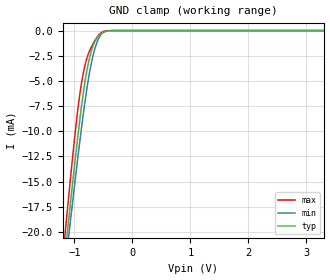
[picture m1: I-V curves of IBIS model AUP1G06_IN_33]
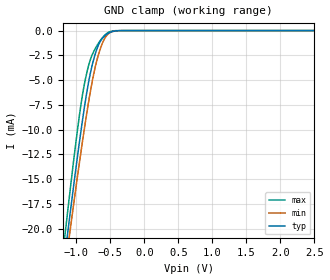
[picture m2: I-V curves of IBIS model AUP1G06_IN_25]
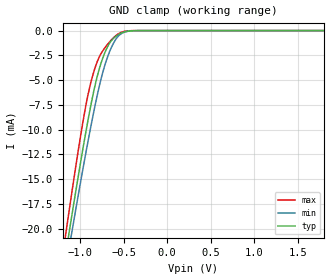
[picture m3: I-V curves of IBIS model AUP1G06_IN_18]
| TEXAS INSTRUMENTS INCORPORATED
| Standard Linear and Logic Group
| IBIS Model of SN74AUP1G06
| Low-Power Single Inverter Buffer/Driver with Open-Drain Output
| This file contains package information for the following:
|  SON 6-pin (DRY) package as [Component] AUP1G06_DRY
|  SON 6-pin (DSF) package as [Component] AUP1G06_DSF
|  SOT 5-pin (DCK) package as [Component] AUP1G06_DCK
|  SOT 5-pin (DBV) package as [Component] AUP1G06_DBV
| This device can be powered at the following Vccs:
|  3.3 volt Vcc
|  2.5 volt Vcc
|  1.8 volt Vcc
|  1.5 volt Vcc
|  1.2 volt Vcc
|  0.8 volt Vcc
| This file provides unique models under the [Model Selector] for each Vcc.
| For operation at a specific Vcc, select the appropriate model after each
| [Model Selector] keyword.
[IBIS Ver]   3.2
[Comment char]  |_char
[File Name]   sn74aup1g06.ibs
[File Rev]   1.1 | x_die
[Date]   April 30,2004
[Source]   Data creted from TI-SPICE simulations at TI-SLL.
[Notes]   The following is an IBIS list for the AUP1G06.
   Please contact sllibis@ti.com with questions and
   comments concerning SLL IBIS models.
   - FILE REV HISTORY
   - 1.1 Release IBIS file on 05/04/04
   - Power clamp data deleted as there is no power-clamp diode.
[Disclaimer] Property of Texas Instruments Incorporated.  Unauthorized
   reproduction and/or distribution is strictly prohibited.
   This product is protected under copyright law.
   Created  2003, (C) Copyright  2003, Texas Instruments
   Incorporated, All Rights Reserved
   UNLESS THERE IS A SIGNED, WRITTEN AGREEMENT TO THE
   CONTRARY, TEXAS INSTRUMENTS (TI) IS PROVIDING THE IBIS
   MODELS  AND WITHOUT ANY WARRANTY, EXPRESSED OR
   IMPLIED.  TI assumes no liability for:
   1) the accuracy of the IBIS models provided to your
   company;
   2) the proper functioning of these IBIS Models in your
   design or for any resulting applications; or
   3) infringement of patents, copyrights or intellectual
   property rights resulting from your use of these IBIS
   models.
   TI provides IBIS Models as a service to our customers.
   You and your company shall not distribute, sell or give
   these models to anyone else without prior written
   permission from TI.
   TI reserves the right to make changes to our products or
   to discontinue any semiconductor product or service
   without notice, and advises our customers to obtain the
   latest version of relevant information to verify, before
   placing orders, that the information being relied on is
   current.
   Please be aware that your receipt and use of the IBIS
   information provided shall serve as acceptance of these
   terms and conditions.  If you do not accept these terms,
   you should return or destroy the IBIS models and any
   other accompanying information immediately.
| Component AUP1G06_DRY 6-pin SON
[Component]   AUP1G06_DRY
[Manufacturer]   Texas Instruments, Inc.
[Package]
|   typ   min   max
R_pkg   2.61E-02   1.03E-03   4.37E-02
L_pkg   2.94E-10   1.45E-11   5.00E-10
C_pkg   1.01E-13   7.41E-14   1.18E-13
[Pin]   signal_name   model_name   R_pin   L_pin   C_pin
1   NC   NC   1.03E-03   1.46E-11   7.41E-14
2   A   AUP1G06_IN   3.24E-02   3.52E-10   1.09E-13
3   GND   GND   3.93E-02   4.44E-10   1.14E-13
4   Y   AUP1G06_OUT   3.93E-02   4.39E-10   1.14E-13
5   NC   NC   1.03E-03   1.45E-11   7.65E-14
6   VCC   POWER   4.37E-02   5.00E-10   1.18E-13
| Component AUP1G06_DSF 6-pin SON
[Component]   AUP1G06_DSF
[Manufacturer]   Texas Instruments, Inc.
[Package]
|   typ   min   max
R_pkg   2.24E-02   1.03E-03   3.70E-02
L_pkg   2.53E-10   1.77E-11   4.23E-10
C_pkg   9.79E-14   7.41E-14   1.13E-13
[Pin]   signal_name   model_name   R_pin   L_pin   C_pin
1   NC   NC   3.06E-03   1.77E-11   7.41E-14
2   A   AUP1G06_IN   2.77E-02   3.06E-10   1.06E-13
3   GND   GND   3.21E-02   3.60E-10   1.08E-13
4   Y   AUP1G06_OUT   3.35E-02   3.75E-10   1.10E-13
5   NC   NC   1.03E-03   3.45E-11   7.65E-14
6   VCC   POWER   3.70E-02   4.23E-10   1.13E-13
| Component AUP1G06_DCK 5-pin SOT
[Component]   AUP1G06_DCK
[Manufacturer]   Texas Instruments, Inc.
[Package]
|   typ   min   max
R_pkg   2.000e-02   1.700e-02   2.500e-02
L_pkg   9.980e-10   8.810e-10   1.069e-09
C_pkg   1.460e-13   1.180e-13   2.050e-13
[Pin]   signal_name   model_name   R_pin   L_pin   C_pin
1   NC   NC   1.900e-02   1.069e-09   1.620e-13
2   A   AUP1G06_IN   1.800e-02   8.810e-10   1.210e-13
3   GND   GND   1.700e-02   1.031e-09   2.050e-13
4   Y   AUP1G06_OUT   2.000e-02   9.600e-10   1.240e-13
5   VCC   POWER   2.500e-02   1.049e-09   1.180e-13
| Component AUP1G06_DBV 5-pin SOT
[Component]   AUP1G06_DBV
[Manufacturer]   Texas Instruments, Inc.
[Package]
|   typ   min   max
R_pkg   2.500e-02   2.100e-02   2.900e-02
L_pkg   1.529e-09   1.312e-09   1.906e-09
C_pkg   1.560e-13   1.100e-13   2.400e-13
[Pin]   signal_name   model_name   R_pin   L_pin   C_pin
1   NC   NC   2.100e-02   1.511e-09   1.440e-13
2   A   AUP1G06_IN   2.300e-02   1.312e-09   1.380e-13
3   GND   GND   2.900e-02   1.906e-09   2.400e-13
4   Y   AUP1G06_OUT   2.600e-02   1.541e-09   1.500e-13
5   VCC   POWER   2.500e-02   1.374e-09   1.100e-13
| Model AUP1G06_IN
[Model Selector]   AUP1G06_IN
AUP1G06_IN_33   3.3 volt Vcc
AUP1G06_IN_25   2.5 volt Vcc
AUP1G06_IN_18   1.8 volt Vcc
AUP1G06_IN_15   1.5 volt Vcc
AUP1G06_IN_12   1.2 volt Vcc
AUP1G06_IN_08   0.8 volt Vcc
| Model AUP1G06_OUT
[Model Selector]   AUP1G06_OUT
AUP1G06_OUT_33   3.3 volt Vcc
AUP1G06_OUT_25   2.5 volt Vcc
AUP1G06_OUT_18   1.8 volt Vcc
AUP1G06_OUT_15   1.5 volt Vcc
AUP1G06_OUT_12   1.2 volt Vcc
AUP1G06_OUT_08   0.8 volt Vcc
| Models and submodels in the file (12): AUP1G06_IN_33 (Input), AUP1G06_IN_25 (Input), AUP1G06_IN_18 (Input), AUP1G06_IN_15 (Input), AUP1G06_IN_12 (Input), AUP1G06_IN_08 (Input), AUP1G06_OUT_33 (Open_drain), AUP1G06_OUT_25 (Open_drain), AUP1G06_OUT_18 (Open_drain), AUP1G06_OUT_15 (Open_drain), AUP1G06_OUT_12 (Open_drain), AUP1G06_OUT_08 (Open_drain)
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[Model]   AUP1G06_IN_33
Model_type  Input
Vinl=0.9
Vinh=2
| variable   typ   min   max
C_comp   1.41pF   1.15pF   1.78pF
[Temperature Range]   40   100   -40
| Ambient temperature   25   85   -40
[Voltage range]   3.3   3   3.6
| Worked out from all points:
|   GND clamp passes 1 mA (typ) near -0.64 V on its own axis
[GND Clamp]
| AUP1G06_IN_33
|   Voltage   I(typ)   I(min)   I(max)
-3.6V     -171.6mA   -163.5mA   -181.1mA
-1.16V    -22.22mA   -23.69mA   -20.18mA
-1.11V    -19.45mA   -21.09mA   -17.19mA
-1.085V   -18.08mA   -19.81mA   -15.71mA
-940mV    -10.5mA    -12.6mA    -7.822mA
-890mV    -8.117mA   -10.26mA   -5.698mA
-835mV    -5.768mA   -7.825mA   -3.925mA
-755mV    -3.153mA   -4.717mA   -2.255mA
-675mV    -1.463mA   -2.419mA   -1.277mA
-595mV    -617.7uA   -945.8uA   -546.7uA
-515mV    -215.4uA   -248.8uA   -134.4uA
3.3V      132.2pA    540.4pA    36.28pA
[Model]   AUP1G06_IN_25
Model_type  Input
Vinl=0.7
Vinh=1.6
| variable   typ   min   max
C_comp   1.44pF   1.20pF   1.77pF
[Temperature Range]   40   100   -40
| Ambient temperature   25   85   -40
[Voltage range]   2.5   2.3   2.7
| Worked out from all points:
|   GND clamp passes 1 mA (typ) near -0.64 V on its own axis
[GND Clamp]
| AUP1G06_IN_25
|   Voltage   I(typ)   I(min)   I(max)
-3.6V     -171.6mA   -163.5mA   -181.1mA
-1.165V   -22.5mA    -23.95mA   -20.48mA
-1.115V   -19.72mA   -21.35mA   -17.49mA
-1.09V    -18.36mA   -20.06mA   -16.01mA
-945mV    -10.75mA   -12.84mA   -8.061mA
-890mV    -8.117mA   -10.26mA   -5.698mA
-835mV    -5.768mA   -7.825mA   -3.925mA
-760mV    -3.287mA   -4.89mA    -2.329mA
-675mV    -1.463mA   -2.419mA   -1.277mA
-595mV    -617.7uA   -945.8uA   -546.7uA
-520mV    -233.1uA   -272.6uA   -149.9uA
2.5V      104.3pA    491.9pA    26.71pA
[Model]   AUP1G06_IN_18
Model_type  Input
Vinl=0.6825
Vinh=1.0725
| variable   typ   min   max
C_comp   1.49pF   1.27pF   1.76pF
[Temperature Range]   40   100   -40
| Ambient temperature   25   85   -40
[Voltage range]   1.8   1.65   1.95
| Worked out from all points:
|   GND clamp passes 1 mA (typ) near -0.64 V on its own axis
[GND Clamp]
| AUP1G06_IN_18
|   Voltage   I(typ)   I(min)   I(max)
-3.6V     -171.6mA   -163.5mA   -181.1mA
-1.16V    -22.22mA   -23.69mA   -20.18mA
-1.135V   -20.83mA   -22.39mA   -18.68mA
-1.11V    -19.45mA   -21.09mA   -17.19mA
-1.09V    -18.36mA   -20.06mA   -16.01mA
-960mV    -11.5mA    -13.57mA   -8.799mA
-850mV    -6.372mA   -8.471mA   -4.359mA
-780mV    -3.86mA    -5.615mA   -2.659mA
-710mV    -2.096mA   -3.313mA   -1.67mA
-625mV    -855.5uA   -1.409mA   -788.9uA
-540mV    -313.2uA   -390uA     -224.9uA
1.8V      83.14pA    451.3pA    18.98pA
